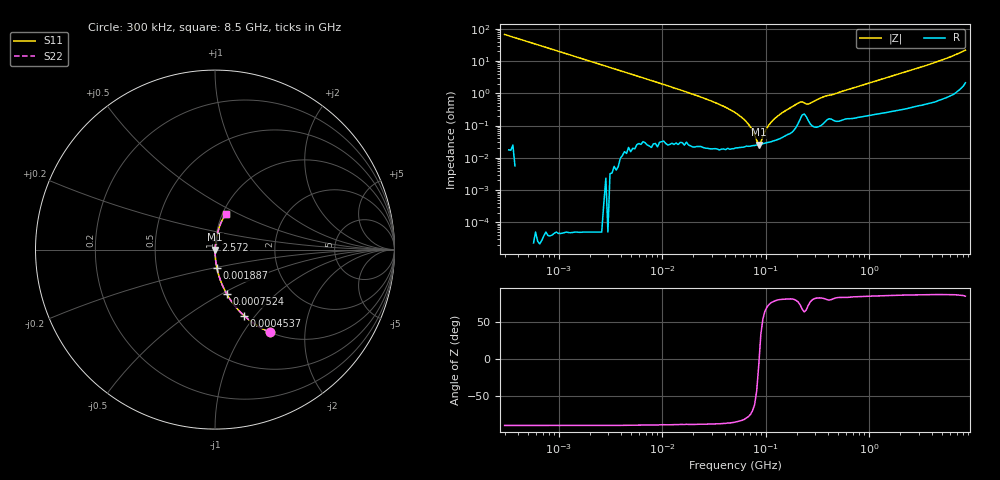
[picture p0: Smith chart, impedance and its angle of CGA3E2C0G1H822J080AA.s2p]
! S-parameter Generated by TDK Corporation
! Copyright(C) 2015 TDK Corporation.
! All Rights Reserved.
! TDK P/N: CGA3E2C0G1H822J080AA (Multilayer Ceramic Chip Capacitors)
! Property: C=8.2nF
! Size(LxWxT): 1.6x0.8x0.8mm, 0.063x0.031x0.031inches
! Model Type: s2p (Touchstone File Format Version 1.0)
! Frequency: DC=Yes Start=0.3MHz Stop=8500MHz 225points Log-sweep
! Note:
! Model Generated on Jun. 23, 2015
! Hash(MD5):
! Port Assignments:
!  1 ---| |--- 2
! Applicable Conditions:
!  Temperature = 25 degC
!  DC Bias Voltage = 0 V
!  Small Signal Operation
! Terms and conditions regarding TDK Simulation Models
! (1)This simulation model is being provided solely for informational purposes. Please refer to the specifications of the products in terms of detailed characteristics of such products.
! (2)In no event shall TDK Corporation of any of its subsidiaries be liable for any loss or damage arising, directly or indirectly,
!  From any information contained in this simulation model, including, but not limited to loss or damages arising from any inaccuracies, omissions or errors in connection with such information.
! (3)Any and all copyrights on this simulation model are owned by TDK Corporation.
!  Duplication or redistribution of this simulation model without prior written permission from TDK Corporation is prohibited.
! (4)This simulation model is subject to any modification or change without any prior notice.
! (5)Neither TDK Corporation nor any of its subsidiaries shall make any warranty, express or implied,
!  Including but not limited to the correctness, implied warranties of merchantability and fitness for a particular purpose with respect to this simulation models.
! (6)The use of this simulation model shall be deemed to have consented to the terms and conditions hereof.
# MHz S MA R 50
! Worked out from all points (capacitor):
!   224 points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, 300 kHz to 8.5 GHz, reference 50 ohm
!   read as one part in series: C = 8.01 nF near 314.1 kHz
!   lowest |Z| = 25.4 mohm at 85.68 MHz (marker M1)
!   series resonance near 86.41 MHz, so ESL is about 420 pH
!   S11 on the Smith chart (normalised r, x): 300 kHz: 1.00, -1.32; 453.7 kHz: 1.00, -0.88; 752.4 kHz: 1.00, -0.53; 1.887 MHz: 1.00, -0.21; 2.572 GHz: 1.01, +0.10; 8.5 GHz: 1.04, +0.43
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0.3  0.5521 -56.5  0.8338 33.5  0.8338 33.5  0.5521 -56.5
0.4537435  0.4014 -66.3  0.9159 23.7  0.9159 23.7  0.4014 -66.3
0.7523683  0.2553 -75.2  0.9669 14.8  0.9669 14.8  0.2553 -75.2
1.72111  0.1144 -83.4  0.9934 6.6  0.9934 6.6  0.1144 -83.4
1.88686  0.1044 -84.0  0.9945 6.0  0.9945 6.0  0.1044 -84.0
9.430415  0.02052 -88.0  0.9995 1.2  0.9995 1.2  0.02052 -88.0
29.76236  0.005753 -87.8  0.9998 0.3  0.9998 0.3  0.005753 -87.8
51.67171  0.002407 -85.0  0.9998 0.1  0.9998 0.1  0.002407 -85.0
68.08408  0.001099 -78.1  0.9998 0.1  0.9998 0.1  0.001099 -78.1
74.64084  0.0006939 -69.9  0.9998 0.0  0.9998 0.0  0.0006939 -69.9
85.6787  0.000253 -8.5  0.9997 0.0  0.9997 0.0  0.000253 -8.5
89.70948  0.0003058 32.7  0.9997 -0.0  0.9997 -0.0  0.0003058 32.7
98.34885  0.0006509 64.1  0.9997 -0.0  0.9997 -0.0  0.0006509 64.1
102.9757  0.0008484 69.8  0.9997 -0.0  0.9997 -0.0  0.0008484 69.8
129.5872  0.001928 79.0  0.9996 -0.1  0.9996 -0.1  0.001928 79.0
214.8731  0.005278 72.6  0.9984 -0.3  0.9984 -0.3  0.005278 72.6
258.2521  0.004617 72.0  0.9986 -0.3  0.9986 -0.3  0.004617 72.0
283.1228  0.005333 79.4  0.999 -0.3  0.999 -0.3  0.005333 79.4
373.0505  0.00804 80.4  0.9987 -0.5  0.9987 -0.5  0.00804 80.4
1551.304  0.03155 83.4  0.9969 -1.8  0.9969 -1.8  0.03155 83.4
2572.272  0.05208 83.1  0.995 -3.0  0.995 -3.0  0.05208 83.1
8500  0.2067 72.5  0.9584 -11.9  0.9584 -11.9  0.2067 72.5
